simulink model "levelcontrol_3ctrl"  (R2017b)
settings: Solver=ode3  StartTime=0.0  StopTime=10.0  FixedStep=0.1  RelTol=1e-3
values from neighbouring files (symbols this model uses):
  d1amplitude = 0.05    [ExamplePIbased.m]    (also in levelcontrol_init3.m; levelcontrol_init4.m; levelcontrol_init5.m; levelcontrol_init6.m)
  d1bias = 0    [ExamplePIbased.m]    (also in levelcontrol_init3.m; levelcontrol_init4.m; levelcontrol_init5.m; levelcontrol_init6.m)
  d1freq = 1    [ExamplePIbased.m]    (also in levelcontrol_init3.m; levelcontrol_init4.m; levelcontrol_init5.m; levelcontrol_init6.m)
  d1phase = 0    [ExamplePIbased.m]    (also in levelcontrol_init3.m; levelcontrol_init4.m; levelcontrol_init5.m; levelcontrol_init6.m)
  d2 = 0.4    [ExamplePIbased.m]    (also in levelcontrol_init3.m = 0.2; levelcontrol_init4.m = 0.2; levelcontrol_init5.m; levelcontrol_init6.m = 0.2)
  d3 = -0.8    [ExamplePIbased.m]    (also in levelcontrol_init3.m = 0.2; levelcontrol_init4.m = 0.2; levelcontrol_init5.m; levelcontrol_init6.m = 0.2)
  d4 = 0.05    [ExamplePIbased.m]    (also in levelcontrol_init3.m = 0.1; levelcontrol_init4.m; levelcontrol_init5.m; levelcontrol_init6.m)
  d5 = -0.9    [ExamplePIbased.m]    (also in levelcontrol_init3.m; levelcontrol_init4.m; levelcontrol_init5.m; levelcontrol_init6.m)
  est = 1 -> use h_est    [levelcontrol_init3.m]    (also in levelcontrol_init4.m; levelcontrol_init5.m; levelcontrol_init6.m)
  eta = 1e0    (= 1)    [levelcontrol_init3.m]    (also in levelcontrol_init4.m; levelcontrol_init5.m; levelcontrol_init6.m)
  h_est_init = 0.4    [levelcontrol_init3.m]    (also in levelcontrol_init4.m; levelcontrol_init5.m; levelcontrol_init6.m)
  h_init = 0.5    [levelcontrol_init3.m]    (also in levelcontrol_init4.m; levelcontrol_init5.m; levelcontrol_init6.m)
  h_set = 0.5    [ExamplePIbased.m]    (also in levelcontrol_init3.m; levelcontrol_init4.m; levelcontrol_init5.m; levelcontrol_init6.m)
  Kc = (1/kprime)*(1/(tau_c+theta))    (= -0.333333333333)    [ExamplePIbased.m]    (also in levelcontrol_init3.m; levelcontrol_init4.m; levelcontrol_init5.m; levelcontrol_init6.m)
  Kcmax = Kcmin    (= -6.66666666667)    [ExamplePIbased.m]    (also in levelcontrol_init3.m = -10; levelcontrol_init4.m; levelcontrol_init5.m; levelcontrol_init6.m)
  Kcmin = f*Kc    (= -6.66666666667)    [ExamplePIbased.m]    (also in levelcontrol_init3.m = -10; levelcontrol_init4.m; levelcontrol_init5.m; levelcontrol_init6.m)
  LEKF = [pEKF(1) pEKF(2); pEKF(2) pEKF(3)]*transpose(C)*REKFinv    [levelcontrol_init3.m]    (also in levelcontrol_init4.m; levelcontrol_init5.m; levelcontrol_init6.m)
  LLSO = eta*[pLSO(1) pLSO(2); pLSO(2) pLSO(3)]*transpose(C)*RLSOinv    [levelcontrol_init3.m]    (also in levelcontrol_init4.m; levelcontrol_init5.m; levelcontrol_init6.m)
  noise_ON = 0    [ExamplePIbased.m]    (also in levelcontrol_init3.m = 1; levelcontrol_init4.m; levelcontrol_init5.m; levelcontrol_init6.m = 1)
  p = 1    [ExamplePIbased.m]    (also in levelcontrol_init3.m; levelcontrol_init4.m; levelcontrol_init5.m; levelcontrol_init6.m)
  Q = [1e-1 0; 0 1e0]    [levelcontrol_init3.m]    (also in levelcontrol_init4.m; levelcontrol_init5.m; levelcontrol_init6.m)
  q_in_est_init = 0.4    [levelcontrol_init3.m]    (also in levelcontrol_init4.m; levelcontrol_init5.m; levelcontrol_init6.m)
  qin0 = 0.5    [ExamplePIbased.m]    (also in levelcontrol_init3.m; levelcontrol_init4.m; levelcontrol_init5.m; levelcontrol_init6.m)
  qout0 = 0.5    [ExamplePIbased.m]    (also in levelcontrol_init3.m; levelcontrol_init4.m; levelcontrol_init5.m; levelcontrol_init6.m)
  s = 2    [levelcontrol_init3.m]    (also in levelcontrol_init4.m = 1; levelcontrol_init5.m = 1; levelcontrol_init6.m = 1; Compressor_script.m = tf('s'))
  sin_ON = 1    [ExamplePIbased.m]    (also in levelcontrol_init3.m; levelcontrol_init4.m = 0; levelcontrol_init5.m; levelcontrol_init6.m)
  t_delay = 2    [levelcontrol_init3.m]    (also in levelcontrol_init4.m; levelcontrol_init5.m; levelcontrol_init6.m)
  tau_c = 3    [ExamplePIbased.m]    (also in levelcontrol_init3.m; levelcontrol_init4.m; levelcontrol_init5.m; levelcontrol_init6.m)
  tauI = 4*(tau_c+theta)    (= 12)    [ExamplePIbased.m]    (also in levelcontrol_init3.m; levelcontrol_init4.m; levelcontrol_init5.m; levelcontrol_init6.m)
  td2 = 30    [ExamplePIbased.m]    (also in levelcontrol_init3.m = 50; levelcontrol_init4.m = 50; levelcontrol_init5.m; levelcontrol_init6.m = 50)
  td3 = 200    [ExamplePIbased.m]    (also in levelcontrol_init3.m = 100; levelcontrol_init4.m = 100; levelcontrol_init5.m; levelcontrol_init6.m = 100)
  td4 = 350    [ExamplePIbased.m]    (also in levelcontrol_init3.m = 150; levelcontrol_init4.m = 150; levelcontrol_init5.m; levelcontrol_init6.m = 150)
  td5 = 300    [ExamplePIbased.m]    (also in levelcontrol_init3.m = 200; levelcontrol_init4.m = 205; levelcontrol_init5.m; levelcontrol_init6.m = 205)
  Umaxsat = Umax-qout0    (= 0.5)    [ExamplePIbased.m]    (also in levelcontrol_init3.m; levelcontrol_init4.m; levelcontrol_init5.m; levelcontrol_init6.m)
  Uminsat = Umin-qout0    (= -0.5)    [ExamplePIbased.m]    (also in levelcontrol_init3.m; levelcontrol_init4.m; levelcontrol_init5.m; levelcontrol_init6.m)
  useEKF = 0    [levelcontrol_init3.m]    (also in levelcontrol_init4.m; levelcontrol_init5.m; levelcontrol_init6.m)
  useLSO = 1    [levelcontrol_init3.m]    (also in levelcontrol_init4.m; levelcontrol_init5.m; levelcontrol_init6.m)
  Ymax = 0.9-offset    (= 0.84)    [ExamplePIbased.m]    (also in levelcontrol_init3.m = 0.9; levelcontrol_init4.m; levelcontrol_init5.m; levelcontrol_init6.m)
  Ymin = 0.1+offset    (= 0.16)    [ExamplePIbased.m]    (also in levelcontrol_init3.m = 0.1; levelcontrol_init4.m; levelcontrol_init5.m; levelcontrol_init6.m)
undefined symbols (not defined in the file or in its folder): Riccati_init, Rinverse, roc, SimpleTank_ODE, tauImax, tauImin
libraries: simulink x5

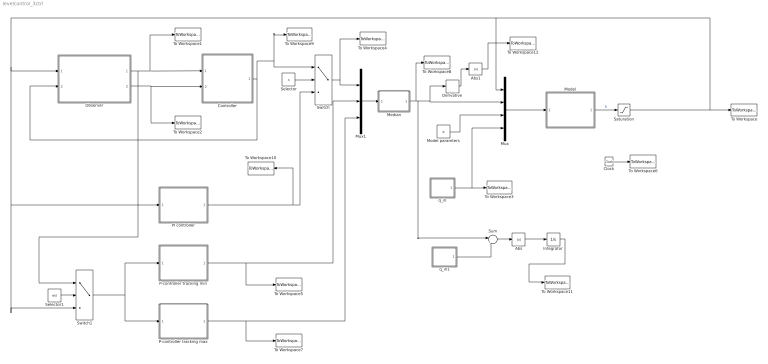
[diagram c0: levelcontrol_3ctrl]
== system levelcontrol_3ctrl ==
  Abs : Abs
  Abs1 : Abs
  Clock : Clock
  Controller : Subsystem
  Derivative : Derivative
  Integrator : Integrator
  Median : MATLAB Function  TreatAsAtomicUnit=on
  Model : Subsystem
  Model paramters : Constant  Value=p
  Mux : Mux
  Mux1 : Mux  Inputs=3
  Observer : Subsystem
  P-controller tracking max : Subsystem
  P-controller tracking min : Subsystem
  PI controller : Subsystem
  Saturation : Saturate  UpperLimit=1  LowerLimit=0
  Selector : Constant  Value=s
  Selector1 : Constant  Value=est
  Sum : Sum  Inputs=|+-
  Switch : Switch  Criteria=u2 > Threshold  Threshold=1.5
  Switch1 : Switch  Criteria=u2 > Threshold  Threshold=0.5
  To Workspace : ToWorkspace  VariableName=h  SaveFormat=Structure With Time  SampleTime=-1
  To Workspace1 : ToWorkspace  VariableName=h_est  SaveFormat=Structure With Time  SampleTime=-1
  To Workspace10 : ToWorkspace  VariableName=q_outPI  SaveFormat=Structure With Time  SampleTime=-1
  To Workspace11 : ToWorkspace  VariableName=IAE_q  SaveFormat=Structure With Time  SampleTime=-1
  To Workspace12 : ToWorkspace  VariableName=derqout  SaveFormat=Structure With Time  SampleTime=-1
  To Workspace2 : ToWorkspace  VariableName=q_in_est  SaveFormat=Structure With Time  SampleTime=-1
  To Workspace3 : ToWorkspace  VariableName=q_in  SaveFormat=Structure With Time  SampleTime=-1
  To Workspace4 : ToWorkspace  VariableName=q_outmid  SaveFormat=Structure With Time  SampleTime=-1
  To Workspace5 : ToWorkspace  VariableName=q_outmin  SaveFormat=Structure With Time  SampleTime=-1
  To Workspace6 : ToWorkspace  VariableName=time  SampleTime=-1
  To Workspace7 : ToWorkspace  VariableName=q_outmax  SaveFormat=Structure With Time  SampleTime=-1
  To Workspace8 : ToWorkspace  VariableName=q_out  SaveFormat=Structure With Time  SampleTime=-1
  To Workspace9 : ToWorkspace  VariableName=q_outObs  SaveFormat=Structure With Time  SampleTime=-1
  q_in : Subsystem
  q_in1 : Subsystem
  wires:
  q_in/1(q_in) -> Mux/4, To Workspace3/1
  Controller/1(q_out) -> Observer/2(q_out), To Workspace9/1, Switch/1
  Observer/2(q_in_est) -> Controller/2(q_in_est2), To Workspace2/1
  Observer/1(h_est) -> Switch1/1, Controller/1(h_est), To Workspace1/1
  Mux/1 -> Model/1(x,u,p,d)
  Model paramters/1 -> Mux/3
  Mux1/1 -> Median/1(u)
  Clock/1 -> To Workspace6/1
  Model/1(h) -> Saturation/1  "h"
  Switch/1 -> To Workspace4/1, Mux1/1
  Selector/1 -> Switch/2
  P-controller tracking min/1(u_min) -> Mux1/2, To Workspace5/1
  P-controller tracking max/1(u_max) -> Mux1/3, To Workspace7/1
  Selector1/1 -> Switch1/2
  Switch1/1 -> P-controller tracking min/1(h), P-controller tracking max/1(h)
  PI controller/1(u_mid) -> Switch/3, To Workspace10/1
  q_in1/1(q_in) -> Sum/2
  Sum/1 -> Abs/1
  Integrator/1 -> To Workspace11/1
  Abs/1 -> Integrator/1
  Saturation/1 -> To Workspace/1, Observer/1(h), Switch1/3, PI controller/1(h), Mux/1
  Median/1(y) -> Sum/1, Derivative/1, Mux/2, To Workspace8/1
  Derivative/1 -> Abs1/1
  Abs1/1 -> To Workspace12/1

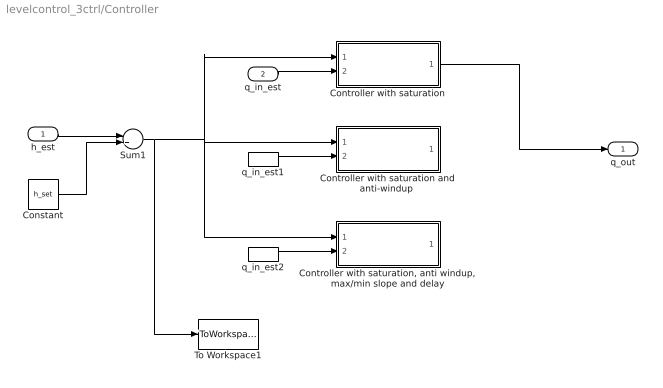
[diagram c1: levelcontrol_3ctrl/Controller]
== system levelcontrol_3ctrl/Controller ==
  h_est : Inport
  q_in_est : Inport  Port=2
  Constant : Constant  Value=h_set
  Controller with saturation : Subsystem
  "Controller with saturation and anti-windup " : Subsystem  Commented=on
  "Controller with saturation, anti windup, max/min slope and delay" : Subsystem  Commented=on
  Sum1 : Sum  Inputs=-+
  To Workspace1 : ToWorkspace  VariableName=error_level  SaveFormat=Structure With Time  SampleTime=-1
  q_in_est1 : InportShadow  Port=2
  q_in_est2 : InportShadow  Port=2
  q_out : Outport
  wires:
  h_est/1 -> Sum1/1
  Sum1/1 -> To Workspace1/1, "Controller with saturation and anti-windup "/1(error_level), "Controller with saturation, anti windup, max/min slope and delay"/1(error_level), Controller with saturation/1(error_level)
  Constant/1 -> Sum1/2
  Controller with saturation/1(u) -> q_out/1
  q_in_est/1 -> Controller with saturation/2(q_in_est)
  q_in_est1/1 -> "Controller with saturation and anti-windup "/2(q_in_est)
  q_in_est2/1 -> "Controller with saturation, anti windup, max/min slope and delay"/2(q_in_est)

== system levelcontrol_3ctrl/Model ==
  x,u,p,d : Inport
  Band-Limited White Noise : simulink/Sources/Band-Limited White Noise  Cov=noise_power  Ts=0.1  seed=[23341]
  Gain : Gain  Gain=noise_ON
  Integrator : Integrator  InitialCondition=h_init
  Sum1 : Sum  Inputs=|++
  Tank model : MATLABFcn  MATLABFcn=SimpleTank_ODE(u(1),u(2),u(3),u(4))  OutputDimensions=1
  h : Outport
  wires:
  Tank model/1 -> Integrator/1
  Sum1/1 -> h/1
  x,u,p,d/1 -> Tank model/1
  Integrator/1 -> Sum1/1
  Band-Limited White Noise/1 -> Gain/1
  Gain/1 -> Sum1/2

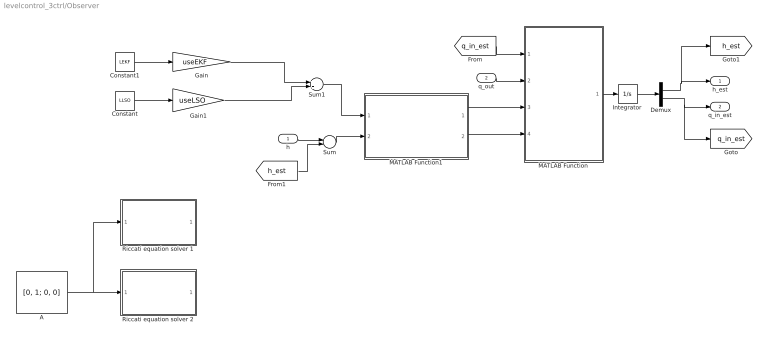
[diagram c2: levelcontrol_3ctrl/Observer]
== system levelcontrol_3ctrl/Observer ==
  h : Inport
  q_out : Inport  Port=2
  A : Constant  Commented=on  Value=[0, 1; 0, 0]
  Constant : Constant  Value=LLSO
  Constant1 : Constant  Value=LEKF
  Demux : Demux  Outputs=2
  Gain : Gain  Gain=useEKF
  Gain1 : Gain  Gain=useLSO
  Integrator : Integrator  InitialCondition=[h_est_init; q_in_est_init]
  MATLAB Function : MATLAB Function  TreatAsAtomicUnit=on
  MATLAB Function1 : MATLAB Function  TreatAsAtomicUnit=on
  Riccati equation solver 1 : Subsystem  Commented=on
  Riccati equation solver 2 : Subsystem  Commented=on
  Sum : Sum  Inputs=+-
  Sum1 : Sum
  h_est : Outport
  q_in_est : Outport  Port=2
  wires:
  A/1 -> Riccati equation solver 1/1(A), Riccati equation solver 2/1(A)
  h/1 -> Sum/1
  MATLAB Function/1(y) -> Integrator/1
  Integrator/1 -> Demux/1
  Demux/1 -> [h_est], h_est/1
  Demux/2 -> [q_in_est], q_in_est/1
  q_out/1 -> MATLAB Function/2(q_out)
  [q_in_est] -> MATLAB Function/1(q_in)
  [h_est] -> Sum/2
  MATLAB Function1/1(Compensation1) -> MATLAB Function/3(Compensation1)
  MATLAB Function1/2(Compensation2) -> MATLAB Function/4(Compensation2)
  Sum/1 -> MATLAB Function1/2(error_h)
  Gain/1 -> Sum1/1
  Constant1/1 -> Gain/1
  Gain1/1 -> Sum1/2
  Constant/1 -> Gain1/1
  Sum1/1 -> MATLAB Function1/1(L)

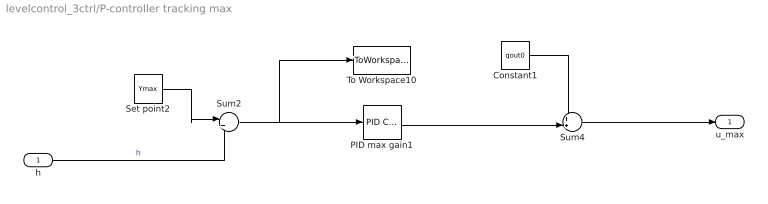
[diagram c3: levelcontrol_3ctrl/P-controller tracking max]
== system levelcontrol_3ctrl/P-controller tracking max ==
  h : Inport
  Constant1 : Constant  Value=qout0
  PID max gain1 : simulink/Continuous/PID Controller  Controller=P  TimeDomain=Continuous-time  SampleTime=-1  IntegratorMethod=Forward Euler  FilterMethod=Forward Euler  Form=Parallel  UseFilter=on  ControllerParametersSource=internal  P=Kcmax  I=Kcmax/tauImax  D=0  N=100  InitialConditionSource=internal  InitialConditionForIntegrator=0  InitialConditionForFilter=0  ExternalReset=none  LimitOutput=on  UpperSaturationLimit=Umaxsat  LowerSaturationLimit=Uminsat  LinearizeAsGain=on  AntiWindupMode=back-calculation  Kb=1  TrackingMode=on  Kt=1  PParamMin=[]  PParamMax=[]  IParamMin=[]  IParamMax=[]  DParamMin=[]  DParamMax=[]  NParamMin=[]  NParamMax=[]  KbParamMin=[]  KbParamMax=[]  KtParamMin=[]  KtParamMax=[]  POutMin=[]  POutMax=[]  IOutMin=[]  IOutMax=[]  DOutMin=[]  DOutMax=[]  NOutMin=[]  NOutMax=[]  KbOutMin=[]  KbOutMax=[]  KtOutMin=[]  KtOutMax=[]  IntegratorOutMin=[]  IntegratorOutMax=[]  FilterOutMin=[]  FilterOutMax=[]  SumOutMin=[]  SumOutMax=[]  SumI1OutMin=[]  SumI1OutMax=[]  SumI2OutMin=[]  SumI2OutMax=[]  SumI3OutMin=[]  SumI3OutMax=[]  SumDOutMin=[]  SumDOutMax=[]  SaturationOutMin=[]  SaturationOutMax=[]  IntegratorContinuousStateAttributes=''  IntegratorStateMustResolveToSignalObject=off  IntegratorRTWStateStorageClass=Auto  FilterContinuousStateAttributes=''  FilterStateMustResolveToSignalObject=off  FilterRTWStateStorageClass=Auto  DifferentiatorICPrevScaledInput=0  DifferentiatorOutMin=[]  DifferentiatorOutMax=[]  InitialConditionSetting=State (most efficient)  FilterDiffOutCoefMin=[]  FilterDiffOutCoefMax=[]  SumDenOutMin=[]  SumDenOutMax=[]  SumNumOutMin=[]  SumNumOutMax=[]  ReciprocalOutMin=[]  ReciprocalOutMax=[]  DivideOutMin=[]  DivideOutMax=[]  TunerSelectOption=Transfer Function Based (PID Tuner App)
  Set point2 : Constant  Value=Ymax
  Sum2 : Sum  Inputs=|+-
  Sum4 : Sum  Inputs=++|
  To Workspace10 : ToWorkspace  VariableName=emax  SampleTime=-1
  u_max : Outport
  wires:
  Set point2/1 -> Sum2/1
  h/1 -> Sum2/2  "h"
  Sum2/1 -> PID max gain1/1, To Workspace10/1
  Sum4/1 -> u_max/1
  Constant1/1 -> Sum4/1
  PID max gain1/1 -> Sum4/2

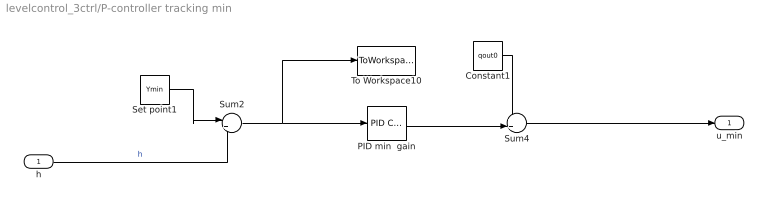
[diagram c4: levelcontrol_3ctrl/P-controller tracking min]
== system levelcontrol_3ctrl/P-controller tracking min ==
  h : Inport
  Constant1 : Constant  Value=qout0
  PID min  gain : simulink/Continuous/PID Controller  Controller=P  TimeDomain=Continuous-time  SampleTime=-1  IntegratorMethod=Forward Euler  FilterMethod=Forward Euler  Form=Parallel  UseFilter=on  ControllerParametersSource=internal  P=Kcmin  I=Kcmin/tauImin  D=0  N=100  InitialConditionSource=internal  InitialConditionForIntegrator=0  InitialConditionForFilter=0  ExternalReset=none  LimitOutput=on  UpperSaturationLimit=Umaxsat  LowerSaturationLimit=Uminsat  LinearizeAsGain=on  AntiWindupMode=back-calculation  Kb=1  TrackingMode=on  Kt=1  PParamMin=[]  PParamMax=[]  IParamMin=[]  IParamMax=[]  DParamMin=[]  DParamMax=[]  NParamMin=[]  NParamMax=[]  KbParamMin=[]  KbParamMax=[]  KtParamMin=[]  KtParamMax=[]  POutMin=[]  POutMax=[]  IOutMin=[]  IOutMax=[]  DOutMin=[]  DOutMax=[]  NOutMin=[]  NOutMax=[]  KbOutMin=[]  KbOutMax=[]  KtOutMin=[]  KtOutMax=[]  IntegratorOutMin=[]  IntegratorOutMax=[]  FilterOutMin=[]  FilterOutMax=[]  SumOutMin=[]  SumOutMax=[]  SumI1OutMin=[]  SumI1OutMax=[]  SumI2OutMin=[]  SumI2OutMax=[]  SumI3OutMin=[]  SumI3OutMax=[]  SumDOutMin=[]  SumDOutMax=[]  SaturationOutMin=[]  SaturationOutMax=[]  IntegratorContinuousStateAttributes=''  IntegratorStateMustResolveToSignalObject=off  IntegratorRTWStateStorageClass=Auto  FilterContinuousStateAttributes=''  FilterStateMustResolveToSignalObject=off  FilterRTWStateStorageClass=Auto  DifferentiatorICPrevScaledInput=0  DifferentiatorOutMin=[]  DifferentiatorOutMax=[]  InitialConditionSetting=State (most efficient)  FilterDiffOutCoefMin=[]  FilterDiffOutCoefMax=[]  SumDenOutMin=[]  SumDenOutMax=[]  SumNumOutMin=[]  SumNumOutMax=[]  ReciprocalOutMin=[]  ReciprocalOutMax=[]  DivideOutMin=[]  DivideOutMax=[]  TunerSelectOption=Transfer Function Based (PID Tuner App)
  Set point1 : Constant  Value=Ymin
  Sum2 : Sum  Inputs=|+-
  Sum4 : Sum  Inputs=++|
  To Workspace10 : ToWorkspace  VariableName=emin1  SampleTime=-1
  u_min : Outport
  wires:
  Set point1/1 -> Sum2/1
  h/1 -> Sum2/2  "h"
  Sum2/1 -> To Workspace10/1, PID min  gain/1
  Constant1/1 -> Sum4/1
  PID min  gain/1 -> Sum4/2
  Sum4/1 -> u_min/1

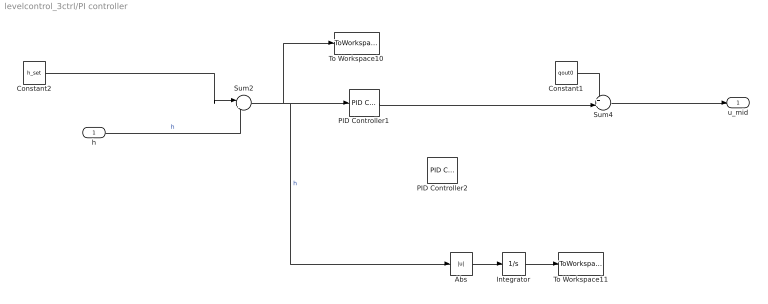
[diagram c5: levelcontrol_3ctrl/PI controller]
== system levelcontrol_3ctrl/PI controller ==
  h : Inport
  Abs : Abs
  Constant1 : Constant  Value=qout0
  Constant2 : Constant  Value=h_set
  Integrator : Integrator
  PID Controller1 : simulink/Continuous/PID Controller  Controller=PI  TimeDomain=Continuous-time  SampleTime=-1  IntegratorMethod=Forward Euler  FilterMethod=Forward Euler  Form=Parallel  UseFilter=on  ControllerParametersSource=internal  P=Kc  I=Kc/tauI  D=0  N=100  InitialConditionSource=internal  InitialConditionForIntegrator=0  InitialConditionForFilter=0  ExternalReset=none  LimitOutput=on  UpperSaturationLimit=Umaxsat  LowerSaturationLimit=Uminsat  LinearizeAsGain=on  AntiWindupMode=none  Kb=1  TrackingMode=off  Kt=1  PParamMin=[]  PParamMax=[]  IParamMin=[]  IParamMax=[]  DParamMin=[]  DParamMax=[]  NParamMin=[]  NParamMax=[]  KbParamMin=[]  KbParamMax=[]  KtParamMin=[]  KtParamMax=[]  POutMin=[]  POutMax=[]  IOutMin=[]  IOutMax=[]  DOutMin=[]  DOutMax=[]  NOutMin=[]  NOutMax=[]  KbOutMin=[]  KbOutMax=[]  KtOutMin=[]  KtOutMax=[]  IntegratorOutMin=[]  IntegratorOutMax=[]  FilterOutMin=[]  FilterOutMax=[]  SumOutMin=[]  SumOutMax=[]  SumI1OutMin=[]  SumI1OutMax=[]  SumI2OutMin=[]  SumI2OutMax=[]  SumI3OutMin=[]  SumI3OutMax=[]  SumDOutMin=[]  SumDOutMax=[]  SaturationOutMin=[]  SaturationOutMax=[]  IntegratorContinuousStateAttributes=''  IntegratorStateMustResolveToSignalObject=off  IntegratorRTWStateStorageClass=Auto  FilterContinuousStateAttributes=''  FilterStateMustResolveToSignalObject=off  FilterRTWStateStorageClass=Auto  DifferentiatorICPrevScaledInput=0  DifferentiatorOutMin=[]  DifferentiatorOutMax=[]  InitialConditionSetting=State (most efficient)  FilterDiffOutCoefMin=[]  FilterDiffOutCoefMax=[]  SumDenOutMin=[]  SumDenOutMax=[]  SumNumOutMin=[]  SumNumOutMax=[]  ReciprocalOutMin=[]  ReciprocalOutMax=[]  DivideOutMin=[]  DivideOutMax=[]  TunerSelectOption=Transfer Function Based (PID Tuner App)
  PID Controller2 : simulink/Continuous/PID Controller  Controller=PI  TimeDomain=Continuous-time  SampleTime=-1  IntegratorMethod=Forward Euler  FilterMethod=Forward Euler  Form=Parallel  UseFilter=on  ControllerParametersSource=internal  P=Kc  I=Kc/tauI  D=0  N=100  InitialConditionSource=internal  InitialConditionForIntegrator=0  InitialConditionForFilter=0  ExternalReset=none  LimitOutput=on  UpperSaturationLimit=Umaxsat  LowerSaturationLimit=Uminsat  LinearizeAsGain=on  AntiWindupMode=none  Kb=1  TrackingMode=off  Kt=1  PParamMin=[]  PParamMax=[]  IParamMin=[]  IParamMax=[]  DParamMin=[]  DParamMax=[]  NParamMin=[]  NParamMax=[]  KbParamMin=[]  KbParamMax=[]  KtParamMin=[]  KtParamMax=[]  POutMin=[]  POutMax=[]  IOutMin=[]  IOutMax=[]  DOutMin=[]  DOutMax=[]  NOutMin=[]  NOutMax=[]  KbOutMin=[]  KbOutMax=[]  KtOutMin=[]  KtOutMax=[]  IntegratorOutMin=[]  IntegratorOutMax=[]  FilterOutMin=[]  FilterOutMax=[]  SumOutMin=[]  SumOutMax=[]  SumI1OutMin=[]  SumI1OutMax=[]  SumI2OutMin=[]  SumI2OutMax=[]  SumI3OutMin=[]  SumI3OutMax=[]  SumDOutMin=[]  SumDOutMax=[]  SaturationOutMin=[]  SaturationOutMax=[]  IntegratorContinuousStateAttributes=''  IntegratorStateMustResolveToSignalObject=off  IntegratorRTWStateStorageClass=Auto  FilterContinuousStateAttributes=''  FilterStateMustResolveToSignalObject=off  FilterRTWStateStorageClass=Auto  DifferentiatorICPrevScaledInput=0  DifferentiatorOutMin=[]  DifferentiatorOutMax=[]  InitialConditionSetting=State (most efficient)  FilterDiffOutCoefMin=[]  FilterDiffOutCoefMax=[]  SumDenOutMin=[]  SumDenOutMax=[]  SumNumOutMin=[]  SumNumOutMax=[]  ReciprocalOutMin=[]  ReciprocalOutMax=[]  DivideOutMin=[]  DivideOutMax=[]  TunerSelectOption=Transfer Function Based (PID Tuner App)
  Sum2 : Sum  Inputs=|+-
  Sum4 : Sum  Inputs=++|
  To Workspace10 : ToWorkspace  VariableName=emid  SampleTime=-1
  To Workspace11 : ToWorkspace  VariableName=IAEmid  SaveFormat=Structure With Time  SampleTime=-1
  u_mid : Outport
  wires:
  h/1 -> Sum2/2  "h"
  Sum4/1 -> u_mid/1
  Constant1/1 -> Sum4/1
  PID Controller1/1 -> Sum4/2
  Constant2/1 -> Sum2/1
  Abs/1 -> Integrator/1
  Sum2/1 -> Abs/1, PID Controller1/1, To Workspace10/1  "h"
  Integrator/1 -> To Workspace11/1

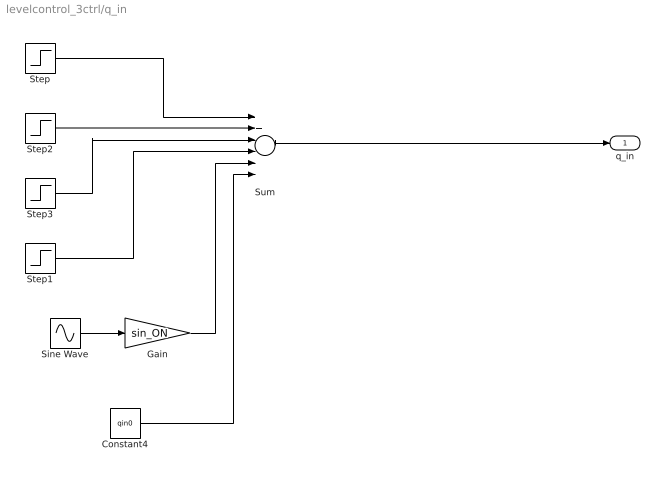
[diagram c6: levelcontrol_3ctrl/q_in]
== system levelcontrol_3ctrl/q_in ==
  Constant4 : Constant  Value=qin0
  Gain : Gain  Gain=sin_ON
  Sine Wave : Sin  Amplitude=d1amplitude  Bias=d1bias  Frequency=d1freq  Phase=d1phase  SampleTime=0
  Step : Step  Time=td2  After=d2  SampleTime=0
  Step1 : Step  Time=td5  After=d5  SampleTime=0
  Step2 : Step  Time=td3  After=d3  SampleTime=0
  Step3 : Step  Time=td4  After=d4  SampleTime=0
  Sum : Sum  Inputs=6
  q_in : Outport
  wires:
  Sum/1 -> q_in/1
  Step/1 -> Sum/1
  Step1/1 -> Sum/4
  Sine Wave/1 -> Gain/1
  Gain/1 -> Sum/5
  Step2/1 -> Sum/2
  Step3/1 -> Sum/3
  Constant4/1 -> Sum/6

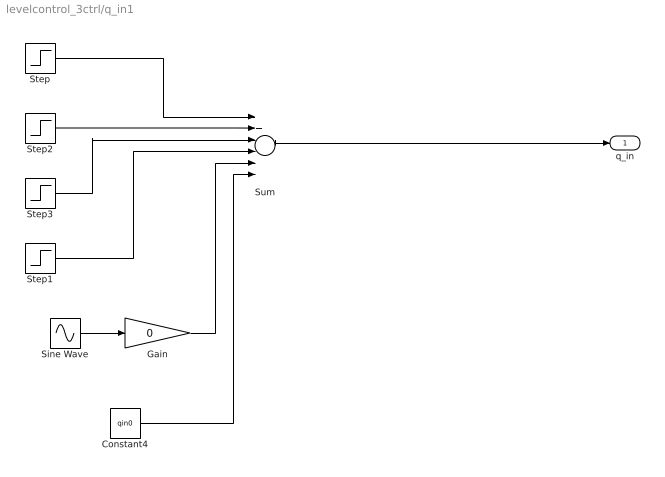
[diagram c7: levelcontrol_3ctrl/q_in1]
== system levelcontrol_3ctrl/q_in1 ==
  Constant4 : Constant  Value=qin0
  Gain : Gain  Gain=0
  Sine Wave : Sin  Amplitude=d1amplitude  Bias=d1bias  Frequency=d1freq  Phase=d1phase  SampleTime=0
  Step : Step  Time=td2  After=d2  SampleTime=0
  Step1 : Step  Time=td5  After=d5  SampleTime=0
  Step2 : Step  Time=td3  After=d3  SampleTime=0
  Step3 : Step  Time=td4  After=d4  SampleTime=0
  Sum : Sum  Inputs=6
  q_in : Outport
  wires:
  Sum/1 -> q_in/1
  Step/1 -> Sum/1
  Step1/1 -> Sum/4
  Sine Wave/1 -> Gain/1
  Gain/1 -> Sum/5
  Step2/1 -> Sum/2
  Step3/1 -> Sum/3
  Constant4/1 -> Sum/6

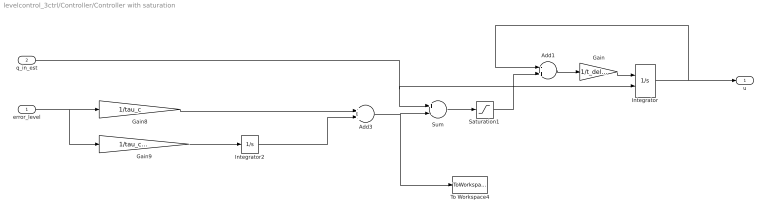
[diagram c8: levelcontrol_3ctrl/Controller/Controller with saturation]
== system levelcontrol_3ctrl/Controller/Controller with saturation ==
  error_level : Inport
  q_in_est : Inport  Port=2
  Add1 : Sum  Inputs=-+
  Add3 : Sum
  Gain : Gain  Gain=1/t_delay
  Gain8 : Gain  Gain=1/tau_c
  Gain9 : Gain  Gain=1/tau_c^2/4
  Integrator : Integrator  InitialConditionSource=external
  Integrator2 : Integrator  UpperSaturationLimit=100  LowerSaturationLimit=0
  Saturation1 : Saturate  UpperLimit=1  LowerLimit=0
  Sum : Sum  Inputs=+-
  To Workspace4 : ToWorkspace  VariableName=pi  SaveFormat=Structure With Time  SampleTime=-1
  u : Outport
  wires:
  Integrator2/1 -> Add3/2
  Gain9/1 -> Integrator2/1
  error_level/1 -> Gain9/1, Gain8/1
  Add3/1 -> To Workspace4/1, Sum/2
  Gain8/1 -> Add3/1
  Sum/1 -> Saturation1/1
  Add1/1 -> Gain/1
  Gain/1 -> Integrator/1
  q_in_est/1 -> Sum/1, Integrator/2
  Integrator/1 -> Add1/1, u/1
  Saturation1/1 -> Add1/2

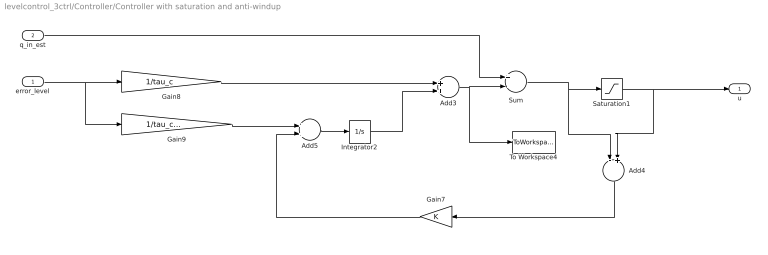
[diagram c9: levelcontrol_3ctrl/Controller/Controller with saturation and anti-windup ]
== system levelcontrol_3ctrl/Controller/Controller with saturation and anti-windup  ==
  error_level : Inport
  q_in_est : Inport  Port=2
  Add3 : Sum
  Add4 : Sum  Inputs=-+
  Add5 : Sum
  Gain7 : Gain
  Gain8 : Gain  Gain=1/tau_c
  Gain9 : Gain  Gain=1/tau_c^2/4
  Integrator2 : Integrator  UpperSaturationLimit=100  LowerSaturationLimit=0
  Saturation1 : Saturate  UpperLimit=1  LowerLimit=0
  Sum : Sum  Inputs=+-
  To Workspace4 : ToWorkspace  VariableName=pi  SaveFormat=Structure With Time  SampleTime=-1
  u : Outport
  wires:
  Integrator2/1 -> Add3/2
  Add5/1 -> Integrator2/1
  Add4/1 -> Gain7/1
  error_level/1 -> Gain9/1, Gain8/1
  Sum/1 -> Saturation1/1, Add4/1
  Gain9/1 -> Add5/1
  Saturation1/1 -> u/1, Add4/2
  Gain7/1 -> Add5/2
  Gain8/1 -> Add3/1
  q_in_est/1 -> Sum/1
  Add3/1 -> To Workspace4/1, Sum/2

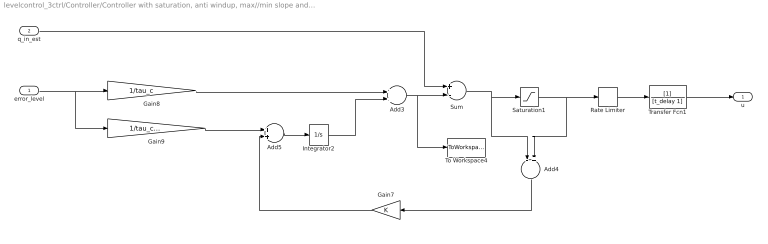
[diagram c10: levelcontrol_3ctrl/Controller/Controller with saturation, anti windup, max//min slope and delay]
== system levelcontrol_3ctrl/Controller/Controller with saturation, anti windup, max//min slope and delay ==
  error_level : Inport
  q_in_est : Inport  Port=2
  Add3 : Sum
  Add4 : Sum  Inputs=-+
  Add5 : Sum
  Gain7 : Gain
  Gain8 : Gain  Gain=1/tau_c
  Gain9 : Gain  Gain=1/tau_c^2/4
  Integrator2 : Integrator  InitialCondition=0.5  UpperSaturationLimit=100  LowerSaturationLimit=0
  Rate Limiter : RateLimiter  RisingSlewLimit=roc  FallingSlewLimit=-roc  SampleTimeMode=inherited
  Saturation1 : Saturate  UpperLimit=1  LowerLimit=0
  Sum : Sum  Inputs=+-
  To Workspace4 : ToWorkspace  VariableName=pi  SaveFormat=Structure With Time  SampleTime=-1
  Transfer Fcn1 : TransferFcn  Denominator=[t_delay 1]
  u : Outport
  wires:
  Integrator2/1 -> Add3/2
  Add5/1 -> Integrator2/1
  Add4/1 -> Gain7/1
  error_level/1 -> Gain9/1, Gain8/1
  Sum/1 -> Saturation1/1, Add4/1
  Gain9/1 -> Add5/1
  Saturation1/1 -> Add4/2, Rate Limiter/1
  Rate Limiter/1 -> Transfer Fcn1/1
  Transfer Fcn1/1 -> u/1
  Gain7/1 -> Add5/2
  Gain8/1 -> Add3/1
  q_in_est/1 -> Sum/1
  Add3/1 -> To Workspace4/1, Sum/2

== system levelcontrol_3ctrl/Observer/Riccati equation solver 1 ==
  A : Inport
  Constant : Constant  Value=Q
  Constant1 : Constant  Value=Rinverse
  Integrator : Integrator  InitialCondition=Riccati_init
  MATLAB Function : MATLAB Function  TreatAsAtomicUnit=on
  MATLAB Function1 : MATLAB Function  TreatAsAtomicUnit=on
  L : Outport
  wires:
  A/1 -> MATLAB Function/1(A)
  MATLAB Function1/1(L) -> L/1, MATLAB Function/2(L)
  Constant/1 -> MATLAB Function/4(Q)
  Constant1/1 -> MATLAB Function1/2(R)
  MATLAB Function/1(dotP) -> Integrator/1
  Integrator/1 -> MATLAB Function1/1(P), MATLAB Function/3(P)

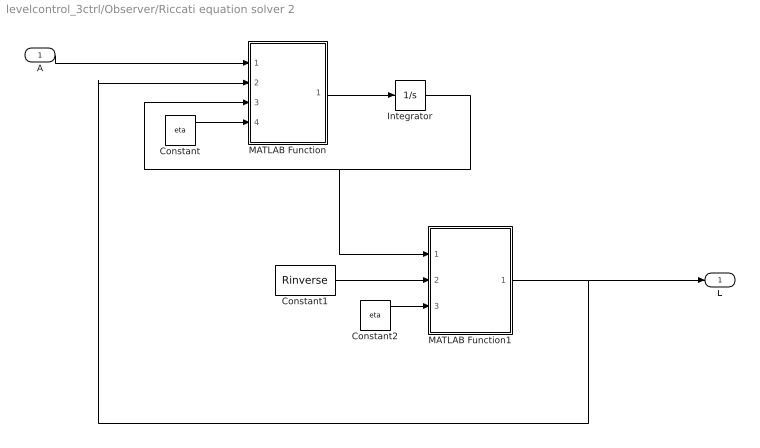
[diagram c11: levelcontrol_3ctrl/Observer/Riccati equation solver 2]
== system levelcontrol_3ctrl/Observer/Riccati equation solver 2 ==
  A : Inport
  Constant : Constant  Value=eta
  Constant1 : Constant  Value=Rinverse
  Constant2 : Constant  Value=eta
  Integrator : Integrator  InitialCondition=Riccati_init
  MATLAB Function : MATLAB Function  TreatAsAtomicUnit=on
  MATLAB Function1 : MATLAB Function  TreatAsAtomicUnit=on
  L : Outport
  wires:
  A/1 -> MATLAB Function/1(A)
  MATLAB Function1/1(L) -> L/1, MATLAB Function/2(L)
  Constant/1 -> MATLAB Function/4(eta)
  Constant1/1 -> MATLAB Function1/2(R)
  Constant2/1 -> MATLAB Function1/3(eta)
  MATLAB Function/1(dotP) -> Integrator/1
  Integrator/1 -> MATLAB Function1/1(P), MATLAB Function/3(P)

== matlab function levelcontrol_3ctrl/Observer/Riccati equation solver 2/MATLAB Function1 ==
function L = fcn(P,R,eta)

L = eta*P*[1; 0]*R;

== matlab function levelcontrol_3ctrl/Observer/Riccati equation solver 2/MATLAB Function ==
function dotP = fcn(A,L,P,eta)

dotP = eta*P+A*P+P*transpose(A) - L*[1 0]*P;

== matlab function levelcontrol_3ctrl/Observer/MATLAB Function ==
function y = fcn(q_in,q_out,Compensation1,Compensation2)

dh = (q_in - q_out) + Compensation1;

dq_in = Compensation2;

y = [dh; dq_in];

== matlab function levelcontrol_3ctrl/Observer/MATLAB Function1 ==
function [Compensation1,Compensation2] = fcn(L,error_h)

Compensation1 = L(1,:)*error_h;
Compensation2 = L(2,:)*error_h;

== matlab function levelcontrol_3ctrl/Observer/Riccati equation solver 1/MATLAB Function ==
function dotP = fcn(A,L,P,Q)

dotP = A*P+P*transpose(A) - L*[1 0]*P + Q;

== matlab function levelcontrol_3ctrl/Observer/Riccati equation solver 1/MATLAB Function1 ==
function L = fcn(P,R)

L = P*[1; 0]*R;

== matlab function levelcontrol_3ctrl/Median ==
function y = fcn(u)

y = median(u);
